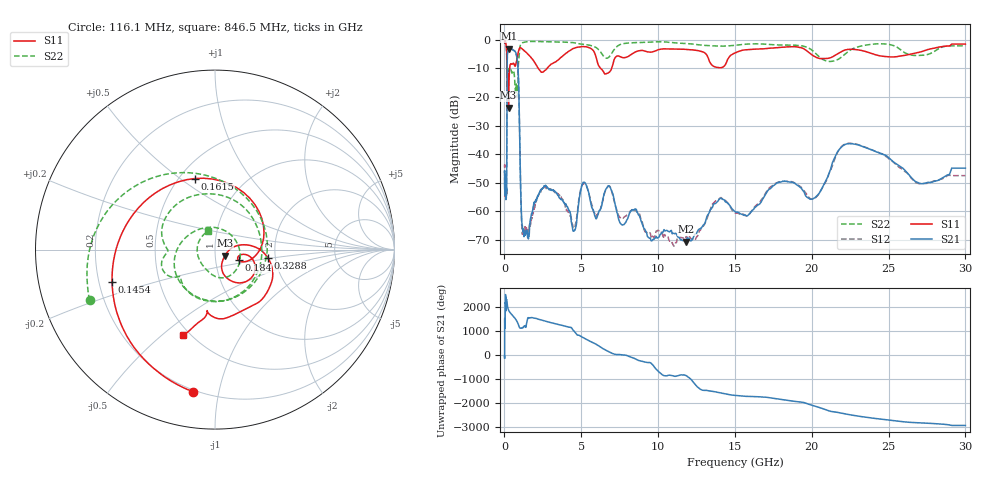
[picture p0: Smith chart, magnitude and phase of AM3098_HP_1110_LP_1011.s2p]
! Date/Time: Thu, Feb 28, 2019 8:46 AM
! Network Analyzer: Agilent Technologies E8364B Rev: A.07.50.67
! Sweep from 0.010 to 30.000 GHz, 1601 Points, Sweep Type: LOG
! Power Supply: 5.022 V, 0.002 A
# Hz S DB R 50
!freq MagS11 AngS11 MagS21 AngS21 MagS12 AngS12 MagS22 AngS22
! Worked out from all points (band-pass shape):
!   1601 points, 10 MHz to 30 GHz, reference 50 ohm
!   highest |S21| = -3.11 dB at 294.5 MHz (marker M1); lowest = -70.6 dB at 11.83 GHz (marker M2)
!   |S21| within 3 dB of the highest: 183.8 MHz to 807.1 MHz (623.4 MHz wide, 126 % of centre)
!   lowest |S11| = -23.8 dB at 265.1 MHz (marker M3), VSWR 1.14, Z = 55.7 - j3.74 ohm
!   |S11| at or under -10 dB: 169.6 MHz to 336.4 MHz (166.8 MHz wide, 65.9 % of centre); 2.196 GHz to 2.777 GHz (581.1 MHz wide, 23.4 % of centre); 6.259 GHz to 6.979 GHz (719.4 MHz wide, 10.9 % of centre)
!   |S22| runs from -20.0 to -0.6 dB; largest |S21 - S12| = 0.011
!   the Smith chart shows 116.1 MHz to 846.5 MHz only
!   S11 on the Smith chart (normalised r, x): 116.1 MHz: 0.19, -0.84; 145.4 MHz: 0.25, -0.14; 161.5 MHz: 0.60, +0.57; 184 MHz: 1.29, -0.16; 328.8 MHz: 1.82, -0.18; 846.5 MHz: 0.46, -0.59
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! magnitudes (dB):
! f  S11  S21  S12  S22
! 10 MHz  -0.3  -46.3  -44.5  -0.6
! 38.04 MHz  -0.3  -51.1  -50.9  -0.8
! 116.1 MHz  -1.9  -54.3  -55.5  -2.5
! 144.7 MHz  -4.3  -50.7  -50.0  -5.4
! 145.4 MHz  -4.4  -49.5  -49.4  -5.6
! 161.5 MHz  -7.7  -23.5  -23.5  -10.6
! 184 MHz  -16.8  -6.1  -6.1  -12.1
! 265.1 MHz  -23.8  -3.2  -3.2  -11.6
! 294.5 MHz  -15.5  -3.1  -3.1  -11.1
! 328.8 MHz  -10.5  -3.2  -3.1  -10.0
! 550.5 MHz  -8.3  -3.6  -3.6  -10.9
! 846.5 MHz  -5.9  -7.7  -7.7  -19.2
! 1.154 GHz  -3.2  -64.9  -66.9  -1.1
! 1.559 GHz  -5.2  -69.6  -66.8  -0.7
! 2.084 GHz  -9.0  -56.3  -55.5  -0.6
! 4.525 GHz  -3.0  -66.9  -65.9  -1.1
! 5.206 GHz  -2.4  -49.8  -50.3  -1.7
! 7.926 GHz  -6.2  -63.5  -61.6  -1.2
! 11.83 GHz  -3.4  -70.6  -68.8  -1.4
! 20.2 GHz  -5.9  -55.2  -55.5  -4.5
! 22.56 GHz  -3.4  -36.3  -36.3  -3.5
! 30 GHz  -1.5  -44.9  -47.5  -2.2
